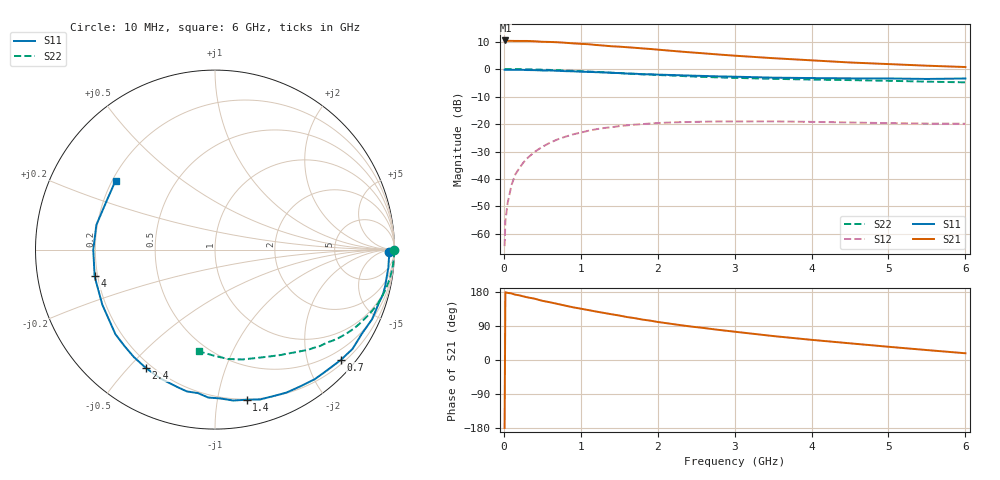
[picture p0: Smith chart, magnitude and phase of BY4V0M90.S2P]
! SIEMENS Small Signal Semiconductors
! BFY420
! Si NPN RF SIEGET Grounded Emitter Transistor in MICRO-X
! VCE = 4 V  IC = 0.9 mA
! Common Emitter S-Parameters:  October  1996
# GHz  S  MA  R  50
!  f  S11  S21  S12  S22
! GHz  MAG  ANG  MAG  ANG  MAG  ANG  MAG  ANG
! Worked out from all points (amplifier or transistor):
!   36 points, 10 MHz to 6 GHz, reference 50 ohm
!   highest |S21| = 10.4 dB at 20 MHz (marker M1)
!   |S21| within 3 dB of that: start of sweep to 1.854 GHz
!   unconditionally stable (mu >= 1): 4.545 GHz to end of sweep
!   at 250 MHz: K = 0.05, MSG = 22.2 dB, |S12| = -34.2 dB
!   at 1.4 GHz: K = 0.18, MSG = 14.7 dB, |S12| = -21.1 dB
!   at 6 GHz: K = 1.36, MAG = 6.8 dB, |S12| = -19.9 dB
!   S11 on the Smith chart (normalised r, x): 10 MHz: 59, -25; 700 MHz: 0.28, -2.63; 1.4 GHz: 0.20, -1.21; 2.4 GHz: 0.18, -0.56; 4 GHz: 0.19, -0.11; 6 GHz: 0.21, +0.30
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0.01  0.9716 -0.7  3.311 -179.4  0.0006 71.0  0.9993 -0.2
0.02  0.9717 -1.2  3.32 178.8  0.0017 77.6  0.9966 -0.5
0.05  0.9702 -3.0  3.269 177.1  0.0037 84.5  0.9976 -1.3
0.1  0.9713 -6.0  3.26 175.7  0.0078 85.5  0.9981 -2.7
0.15  0.9688 -8.9  3.254 172.3  0.0122 82.0  0.9956 -4.0
0.25  0.9688 -15.0  3.252 168.1  0.0196 79.7  0.9923 -6.7
0.4  0.9573 -23.9  3.211 161.8  0.0312 75.5  0.9833 -10.7
0.5  0.9432 -29.7  3.142 156.2  0.0385 72.3  0.9755 -13.3
0.7  0.9324 -41.3  3.079 147.9  0.0527 65.6  0.956 -18.4
0.9  0.9112 -52.4  2.939 139.1  0.0649 58.4  0.9293 -23.1
1.1  0.8907 -63.4  2.835 131.7  0.0756 52.7  0.9023 -27.6
1.4  0.8548 -78.1  2.602 120.7  0.0876 44.3  0.8605 -33.7
1.6  0.8297 -88.0  2.502 113.4  0.0947 38.9  0.8309 -37.5
1.8  0.8053 -96.7  2.38 106.7  0.0998 34.7  0.805 -40.7
2.2  0.7794 -113.2  2.139 94.7  0.1073 26.4  0.7621 -47.1
2.4  0.7636 -120.3  2.03 89.1  0.109 23.2  0.7395 -50.0
2.8  0.7366 -133.4  1.839 79.3  0.1115 17.1  0.7051 -55.3
3.5  0.6988 -154.0  1.58 63.2  0.1117 9.7  0.6655 -63.7
4  0.687 -167.5  1.444 53.2  0.1096 6.0  0.6444 -69.8
4.5  0.6782 -179.9  1.319 44.0  0.1068 3.3  0.6307 -76.1
5.5  0.6619 156.2  1.153 26.2  0.1021 2.3  0.591 -90.6
6  0.6744 145.2  1.091 17.8  0.1014 3.7  0.574 -98.8
